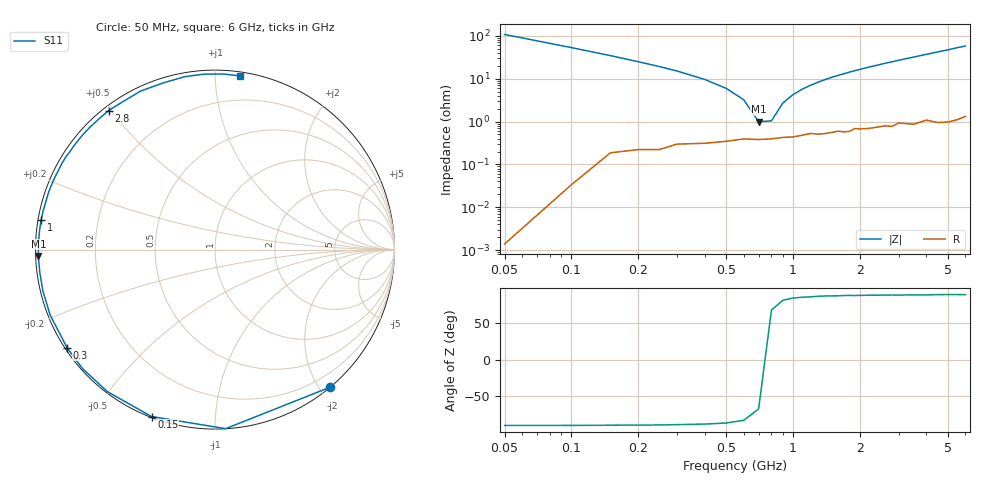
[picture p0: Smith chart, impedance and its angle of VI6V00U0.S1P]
! Infineon Technologies  Discrete & RF Semiconductors
! BB 804
! Si Tuning Diode in SOT23
! VR = 6 V
! S-Parameters:  July  1999
# GHz  S  MA  R  50
!  f  S11
! GHz  MAG  ANG
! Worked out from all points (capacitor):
!   34 points, 50 MHz to 6 GHz, reference 50 ohm
!   read as one part to ground: C = 29.5 pF near 50 MHz
!   lowest |Z| = 992 mohm at 700 MHz (marker M1)
!   series resonance near 748.8 MHz, so ESL is about 1.5 nH
!   S11 on the Smith chart (normalised r, x): 50 MHz: 0.00, -2.14; 150 MHz: 0.00, -0.69; 300 MHz: 0.01, -0.30; 1 GHz: 0.01, +0.08; 2.8 GHz: 0.02, +0.49; 6 GHz: 0.03, +1.15
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0.05  1 -50.0
0.1  0.9994 -86.6
0.15  0.995 -110.8
0.2  0.9929 -127.1
0.25  0.9923 -138.1
0.3  0.9891 -146.5
0.4  0.9881 -158.3
0.5  0.9865 -166.5
0.6  0.9845 -172.7
0.7  0.9849 -177.9
0.8  0.9843 177.8
0.9  0.9832 173.9
1  0.9827 170.4
1.1  0.9813 167.1
1.3  0.9804 161.2
1.6  0.9777 153.2
1.9  0.9752 145.9
2.2  0.976 139.2
2.4  0.9749 135.3
2.6  0.9741 131.0
2.8  0.9755 127.4
3  0.9716 123.5
3.5  0.9757 115.1
4  0.9725 107.1
4.5  0.9779 100.0
5  0.9795 93.7
5.5  0.9794 87.1
6  0.9776 81.9
